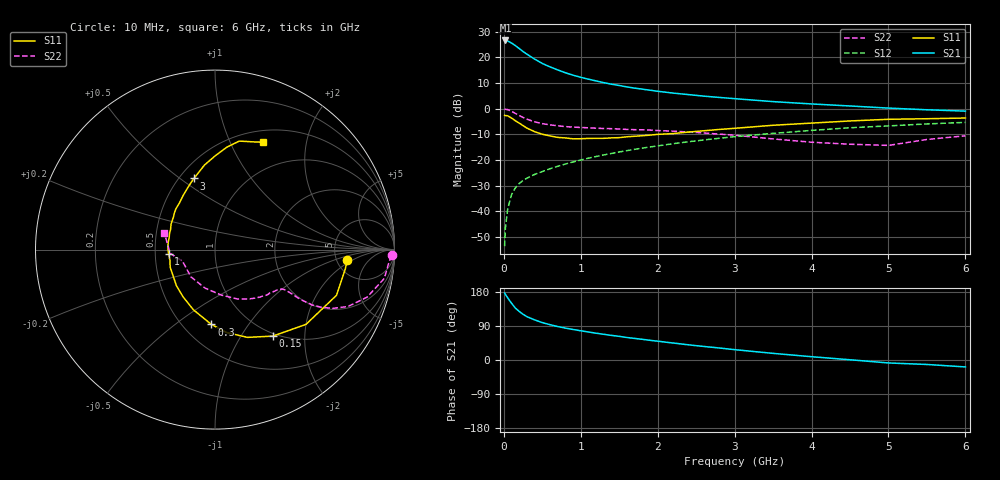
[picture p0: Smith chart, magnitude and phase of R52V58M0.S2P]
! SIEMENS Small Signal Semiconductors
! BFR183
! Si NPN RF Bipolar Junction Transistor in SOT23
! VCE = 2.5 V  IC = 8 mA
! Common Emitter S-Parameters:  May  1996
# GHz  S  MA  R  50
!  f  S11  S21  S12  S22
! GHz  MAG  ANG  MAG  ANG  MAG  ANG  MAG  ANG
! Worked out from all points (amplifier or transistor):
!   36 points, 10 MHz to 6 GHz, reference 50 ohm
!   highest |S21| = 26.5 dB at 20 MHz (marker M1)
!   |S21| within 3 dB of that: start of sweep to 193.6 MHz
!   unconditionally stable (mu >= 1): 827.9 MHz to 2.57 GHz
!   at 250 MHz: K = 0.56, MSG = 25.1 dB, |S12| = -28.0 dB
!   at 1.4 GHz: K = 1.06, MAG = 12.0 dB, |S12| = -17.5 dB
!   at 6 GHz: K = 0.89, MSG = 2.2 dB, |S12| = -5.4 dB
!   lowest NFmin = 1.30 dB at 450 MHz
!   S11 on the Smith chart (normalised r, x): 10 MHz: 6.28, -1.58; 150 MHz: 0.96, -1.39; 300 MHz: 0.68, -0.69; 1 GHz: 0.59, -0.03; 3 GHz: 0.59, +0.56; 6 GHz: 0.64, +1.34
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0.01  0.7399 -4.4  21.1 176.8  0.0021 90.0  0.9848 -1.9
0.02  0.7339 -8.5  21.22 173.3  0.0047 87.3  0.9728 -3.9
0.05  0.7234 -20.6  20.75 163.9  0.0111 80.2  0.9566 -9.7
0.1  0.6562 -39.4  18.9 149.8  0.0211 72.5  0.8875 -17.4
0.15  0.5799 -56.2  16.84 137.1  0.0287 66.5  0.8053 -23.2
0.2  0.5214 -69.7  14.77 128.1  0.0349 63.6  0.7334 -26.5
0.25  0.4662 -82.1  12.92 120.5  0.04 60.9  0.6725 -28.5
0.3  0.4173 -92.8  11.46 114.4  0.0442 60.4  0.6229 -29.7
0.4  0.3556 -110.0  9.205 105.9  0.0523 60.0  0.5529 -30.2
0.5  0.317 -124.4  7.575 98.7  0.0595 60.8  0.5096 -30.1
0.6  0.2942 -137.0  6.492 93.2  0.0676 61.2  0.4832 -29.9
0.7  0.2754 -148.0  5.666 88.3  0.0753 62.3  0.4629 -29.9
0.8  0.2685 -158.3  4.993 84.2  0.0834 62.6  0.4466 -30.0
1  0.2592 -174.6  4.071 77.1  0.0998 63.4  0.4297 -30.8
1.1  0.263 177.9  3.74 73.9  0.1084 63.3  0.4227 -31.8
1.6  0.2832 149.9  2.646 59.4  0.1521 61.7  0.3937 -37.1
2.2  0.3268 127.3  2.004 44.8  0.2075 57.6  0.3638 -46.7
3  0.4133 106.5  1.562 27.3  0.2846 49.6  0.3039 -65.1
3.5  0.4741 97.2  1.368 17.5  0.3297 43.5  0.257 -81.6
4.5  0.5752 83.3  1.125 0.6  0.4242 31.3  0.2026 -131.5
5.5  0.6355 70.9  0.949 -11.8  0.5031 19.1  0.2508 -175.2
6  0.6556 65.8  0.893 -18.3  0.5399 11.2  0.2954 162.3
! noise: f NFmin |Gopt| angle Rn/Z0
0.45  1.3  0.17  43  0.21
0.9  1.35  0.21  115  0.2
1.8  2.05  0.33  -177  0.14
